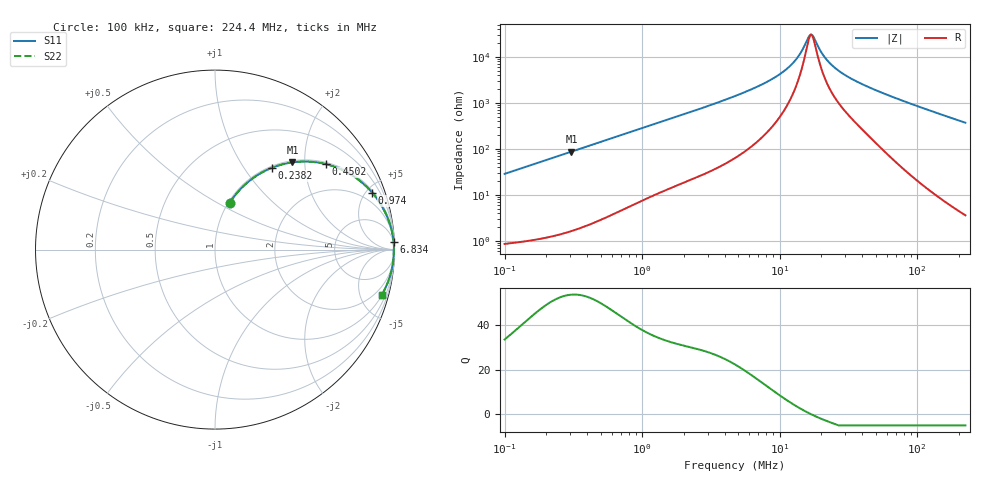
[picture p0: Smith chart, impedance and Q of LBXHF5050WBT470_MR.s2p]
! LBXHF5050WBT470_MR  S-PARAMETER MODEL  ( General Type )
! Model Generated by TAIYO YUDEN Corporation (http://www.ty-top.com)
! Version 1.0
! TAIYO YUDEN Control No. 210719NI43SB-FBB
! Copyright(c) 2021 TAIYO YUDEN CO.,LTD. All Rights Reserved.
! Product Description (link to TY-COMPAS)
! https://ds.yuden.co.jp/TYCOMPAS/or/detail?pn=LBXHF5050WBT470MMR&u=M
! Products Name : Inductors
! Characteristics :
!  Inductance : 47 uH , SRF(min) : 12 MHz , DC Resistance(max) : 0.52 Ohm
!  Rated Current : Saturation :730 mA , Temp Rise : 580 mA
!  Case Size : 5.0 x 5.0 / 0.197 x 0.197 [mm/inch] , Thickness : 2.2 / 0.087 [mm/inch]
!  (Conditions: Temperature = 25 degC , DC Bias Current/Voltage = 0A / 0V)
! External Node Assignments :
!  1  o---GGG---o  2
! GND o---------o GND
! Frequency Range : 0.1MHz  -  224.402193MHz  [ 402 STEP ]
# MHz S RI R 50
! Freq[MHz].  S11 Real  S11 Imag  S21 Real  S21 Imag  S12 Real  S12 Imag  S22 Real  S22 Imag
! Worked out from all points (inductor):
!   401 points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, 100 kHz to 224.4 MHz, reference 50 ohm
!   read as one part in series: L = 45.3 uH near 103.9 kHz
!   highest Q = 53.7 at 306.1 kHz (marker M1), where L = 45.1 uH
!   self-resonance near 16.92 MHz
!   S11 on the Smith chart (normalised r, x): 100 kHz: 1.02, +0.57; 238.2 kHz: 1.03, +1.35; 450.2 kHz: 1.05, +2.55; 974 kHz: 1.14, +5.49; 6.834 MHz: 4, +45; 224.4 MHz: 1.07, -7.40
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0.1  0.0819 0.2597  0.9181 -0.2597  0.9181 -0.2597  0.0819 0.2597
0.155842  0.1698 0.3642  0.8302 -0.3642  0.8302 -0.3642  0.1698 0.3642
0.238227  0.3172 0.4558  0.6828 -0.4558  0.6828 -0.4558  0.3172 0.4558
0.306125  0.4312 0.486  0.5688 -0.486  0.5688 -0.486  0.4312 0.486
0.364164  0.5156 0.4905  0.4844 -0.4905  0.4844 -0.4905  0.5156 0.4905
0.450246  0.617 0.4765  0.383 -0.4765  0.383 -0.4765  0.617 0.4765
0.662219  0.7728 0.408  0.2272 -0.408  0.2272 -0.408  0.7728 0.408
0.973987  0.8764 0.3163  0.1236 -0.3163  0.1236 -0.3163  0.8764 0.3163
1.326154  0.9266 0.2466  0.0734 -0.2466  0.0734 -0.2466  0.9266 0.2466
4.737111  0.9919 0.07  0.0081 -0.07  0.0081 -0.07  0.9919 0.07
6.834195  0.9952 0.0443  0.00477 -0.0443  0.00477 -0.0443  0.9952 0.0443
9.305258  0.9965 0.0271  0.00349 -0.0271  0.00349 -0.0271  0.9965 0.0271
11.72895  0.9969 0.016  0.0031 -0.016  0.0031 -0.016  0.9969 0.016
13.95267  0.9969 0.00832  0.00305 -0.00832  0.00305 -0.00832  0.9969 0.00832
16.28088  0.9968 0.00176  0.00317 -0.00176  0.00317 -0.00176  0.9968 0.00176
17.25085  0.9968 -0.000664  0.00324 0.000664  0.00324 0.000664  0.9968 -0.000664
21.32867  0.9963 -0.00951  0.00366 0.00951  0.00366 0.00951  0.9963 -0.00951
26.37042  0.9958 -0.0185  0.00423 0.0185  0.00423 0.0185  0.9958 -0.0185
36.6046  0.9948 -0.034  0.00522 0.034  0.00522 0.034  0.9948 -0.034
62.8214  0.9919 -0.0687  0.0081 0.0687  0.0081 0.0687  0.9919 -0.0687
121.0445  0.9775 -0.1395  0.0225 0.1395  0.0225 0.1395  0.9775 -0.1395
224.4022  0.9299 -0.2506  0.0701 0.2506  0.0701 0.2506  0.9299 -0.2506
